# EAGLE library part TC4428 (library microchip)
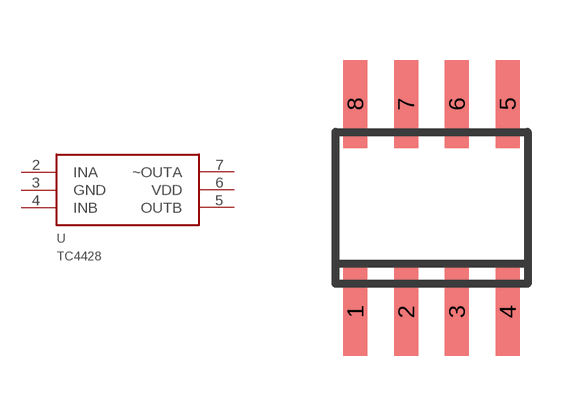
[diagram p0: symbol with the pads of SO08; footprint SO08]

Designator prefix U

## TC4428  [SO08]
2  INA
3  GND
4  INB
5  OUTB
6  VDD
7  ~OUTA

## Footprint SO08 (pad centres in mm)
Small Outline Package
smd 0.6 x 2.2: 1 -1.905,-2.6; 2 -0.635,-2.6; 3 0.635,-2.6; 4 1.905,-2.6; 5 1.905,2.6; 6 0.635,2.6; 7 -0.635,2.6; 8 -1.905,2.6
